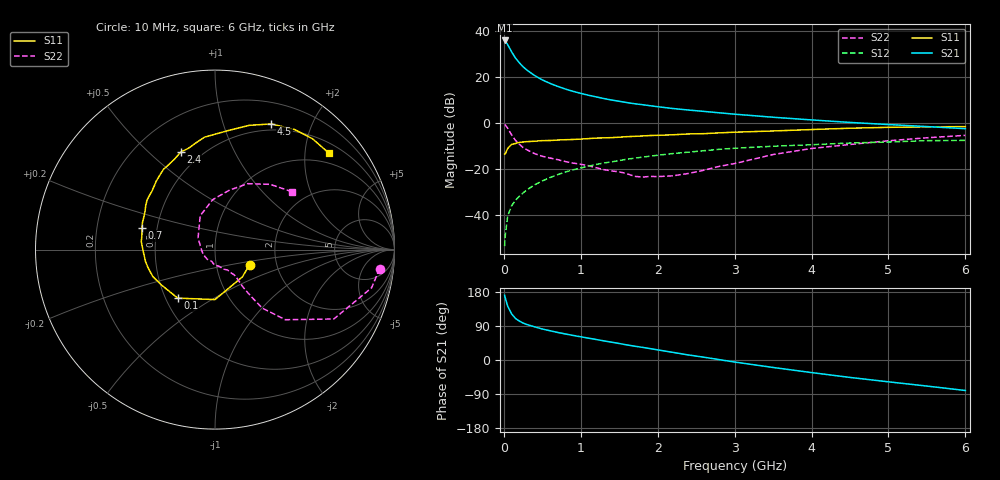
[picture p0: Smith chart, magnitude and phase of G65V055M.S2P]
! SIEMENS Small Signal Semiconductors
! BFG193
! Si NPN RF Bipolar Junction Transistor in SOT223
! VCE = 5 V  IC = 55 mA
! Common Emitter S-Parameters:  August  1996
# GHz  S  MA  R  50
!  f  S11  S21  S12  S22
! GHz  MAG  ANG  MAG  ANG  MAG  ANG  MAG  ANG
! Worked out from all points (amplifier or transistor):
!   36 points, 10 MHz to 6 GHz, reference 50 ohm
!   highest |S21| = 35.8 dB at 10 MHz (marker M1)
!   |S21| within 3 dB of that: start of sweep to 69.17 MHz
!   unconditionally stable (mu >= 1): 428.6 MHz to 2.33 GHz
!   at 250 MHz: K = 0.92, MSG = 27.4 dB, |S12| = -30.4 dB
!   at 1.4 GHz: K = 1.04, MAG = 12.1 dB, |S12| = -16.9 dB
!   at 6 GHz: K = 0.89, MSG = 2.5 dB, |S12| = -7.6 dB
!   S11 on the Smith chart (normalised r, x): 10 MHz: 1.45, -0.25; 100 MHz: 0.58, -0.35; 700 MHz: 0.41, +0.12; 2.4 GHz: 0.39, +0.63; 4.5 GHz: 0.43, +1.46; 6 GHz: 0.73, +2.54
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0.01  0.2103 -23.3  61.93 170.8  0.0021 87.3  0.9232 -6.6
0.02  0.2154 -44.9  59.65 163.0  0.0038 74.9  0.8982 -13.7
0.05  0.2783 -90.0  50.16 141.9  0.0095 72.2  0.7665 -30.3
0.1  0.3409 -127.5  35.32 122.1  0.0157 68.4  0.5535 -44.9
0.15  0.3575 -146.5  25.9 109.8  0.0208 67.3  0.4206 -51.0
0.2  0.3774 -156.6  20.39 102.9  0.0253 68.5  0.3463 -52.1
0.25  0.3859 -164.4  16.62 97.5  0.0302 69.1  0.292 -52.9
0.3  0.3927 -170.1  14.06 93.6  0.0351 69.7  0.2609 -53.2
0.4  0.4001 -178.6  10.71 87.5  0.0452 69.7  0.2151 -52.7
0.5  0.413 173.9  8.6 81.8  0.0549 69.0  0.1886 -52.2
0.6  0.415 168.7  7.229 77.2  0.0651 68.1  0.1729 -53.2
0.7  0.4249 163.5  6.227 72.7  0.0752 66.5  0.1591 -55.2
0.9  0.4368 154.8  4.858 64.8  0.0956 63.0  0.1341 -58.2
1.1  0.4566 147.8  3.996 57.7  0.1149 59.4  0.1176 -67.3
1.3  0.4736 140.7  3.392 50.5  0.1343 55.4  0.0967 -75.4
1.6  0.5034 130.4  2.765 39.8  0.1625 48.6  0.0789 -96.6
2.2  0.5532 113.9  2.055 20.1  0.2162 35.0  0.071 -161.1
2.4  0.5761 109.3  1.906 13.3  0.2321 30.7  0.0799 172.4
3.5  0.6686 83.4  1.329 -19.7  0.3116 3.7  0.2059 113.6
4.5  0.7677 65.8  1.025 -46.0  0.3661 -16.2  0.3402 76.5
5.5  0.8226 48.7  0.833 -68.8  0.4118 -39.6  0.476 49.8
6  0.8314 40.4  0.751 -80.5  0.4175 -53.0  0.537 36.9
